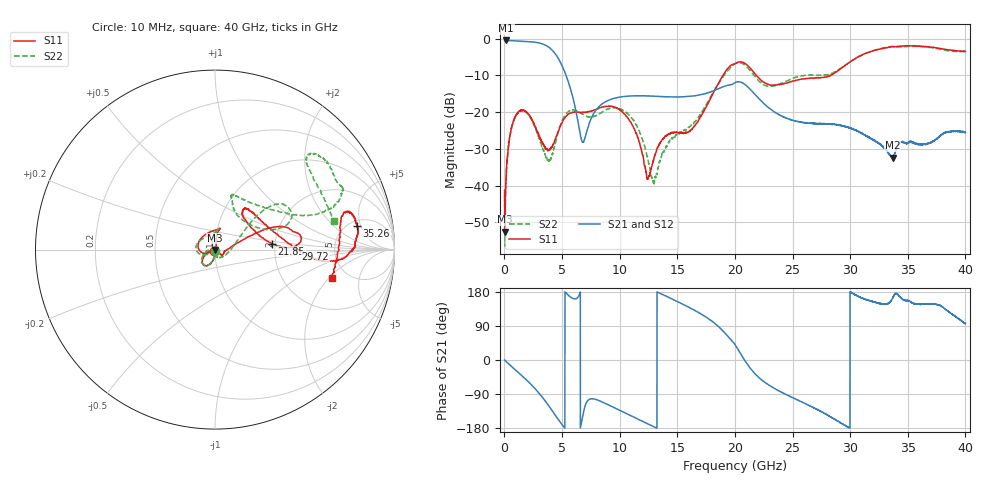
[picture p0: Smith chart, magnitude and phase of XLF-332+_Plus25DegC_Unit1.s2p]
!Created: 10-12-2015 at 09:06:21
!MODEL: XLF-332+
!S/N: Unit 1
# MHZ S DB R 50
!Frequency  S11 dB  S11 DEG  S21 dB  S21 DEG  S12 dB  S12 DEG  S22 dB  S22 DEG
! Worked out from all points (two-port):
!   4000 points, 10 MHz to 40 GHz, reference 50 ohm
!   highest |S21| = -0.45 dB at 140 MHz (marker M1); lowest = -32.4 dB at 33.7 GHz (marker M2)
!   |S21| within 3 dB of the highest: start of sweep to 4.244 GHz
!   lowest |S11| = -52.6 dB at 40 MHz (marker M3), VSWR 1.00, Z = 49.8 - j0.15 ohm
!   |S11| at or under -10 dB: start of sweep to 18.95 GHz; 21.87 GHz to 28.23 GHz (6.358 GHz wide, 25.4 % of centre); 28.25097 GHz to 28.28467 GHz (33.7 MHz wide, 0.119 % of centre)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
!   |S22| runs from -56.5 to -2.0 dB; largest |S21 - S12| = 0.0042
!   S11 on the Smith chart (normalised r, x): 10 MHz: 0.99, -0.01; 21.85 GHz: 1.92, +0.14; 29.72 GHz: 2.64, +0.03; 35.26 GHz: 5.88, +4.27; 40 GHz: 3.78, -2.19
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10  -41.30 -124.1  -0.51 0.0  -0.49 -0.2  -42.77 -103.6
40  -52.60 -140.2  -0.46 -1.2  -0.46 -1.1  -46.49 -113.7
140  -37.64 -97.5  -0.45 -4.2  -0.47 -4.1  -38.14 -93.4
500  -26.04 -98.4  -0.50 -14.0  -0.50 -14.1  -26.00 -98.8
1100  -20.43 -113.8  -0.60 -30.3  -0.59 -30.3  -20.42 -114.4
2900  -25.58 -155.3  -1.06 -84.0  -1.05 -84.0  -26.15 -168.0
3780  -30.38 -159.9  -2.15 -118.1  -2.15 -118.1  -32.94 -170.5
4390  -27.49 -152.6  -4.02 -144.9  -4.02 -144.9  -28.79 -146.9
5380  -21.01 -179.4  -10.29 175.5  -10.29 175.5  -20.34 -169.2
6680  -20.08 128.8  -27.51 -167.2  -27.54 -166.9  -20.34 147.7
10300  -20.14 80.7  -15.78 -137.2  -15.76 -137.1  -19.55 84.9
12450  -38.02 17.9  -15.59 -168.6  -15.59 -168.6  -32.87 129.3
13340  -29.40 -41.1  -15.72 178.3  -15.70 178.5  -35.08 -114.4
16260  -24.69 -6.2  -15.64 134.9  -15.64 134.8  -23.47 -24.1
20010  -6.78 12.3  -11.94 40.7  -11.96 40.4  -6.79 33.2
21850  -9.94 5.9  -15.54 -39.8  -15.53 -40.1  -10.74 23.1
26670  -10.73 50.0  -23.06 -123.4  -23.08 -123.8  -9.86 71.2
29720  -6.91 0.6  -24.09 -175.7  -24.01 -175.9  -6.88 26.4
33340  -2.32 0.2  -31.18 150.0  -31.31 148.6  -2.18 24.3
33700  -2.16 1.3  -32.44 163.7  -32.26 163.9  -2.08 25.9
35260  -1.93 9.4  -27.94 152.2  -28.10 151.4  -2.04 36.2
40000  -3.44 -13.6  -25.49 96.5  -25.64 94.6  -3.28 13.5
